VAR_GLOBAL
	(* error monitoring *)
	fbErrHist			: FB_HRErrHist;
	
	(* signal properties *)
	cCarrierFrequency		: LREAL 	:= 513.0;									// Frequency of carrier signal [Hz]
	cCarrierAmplitude		: LREAL 	:= 10.0;                     				// Amplitude of carrier signal [V]
	cDefectFrequency		: LREAL 	:= 20 * cResolution;          				// Frequency of peaks [Hz]
	cDefectAmplitude		: LREAL 	:= 1.0;                     				// Scaling of peaks with exponential decay [1]
	cDefectDutyCycle		: UINT		:= 50;                      				// Percentage of full period for peak to fall below tolerance (1E-4) [%]
	cShockFrequency			: LREAL 	:= 213 * cResolution;              			// Frequency of shock [Hz]
	cShockAmplitude			: LREAL 	:= 20.0;                     				// Amplidute of shock [V]
	
END_VAR
